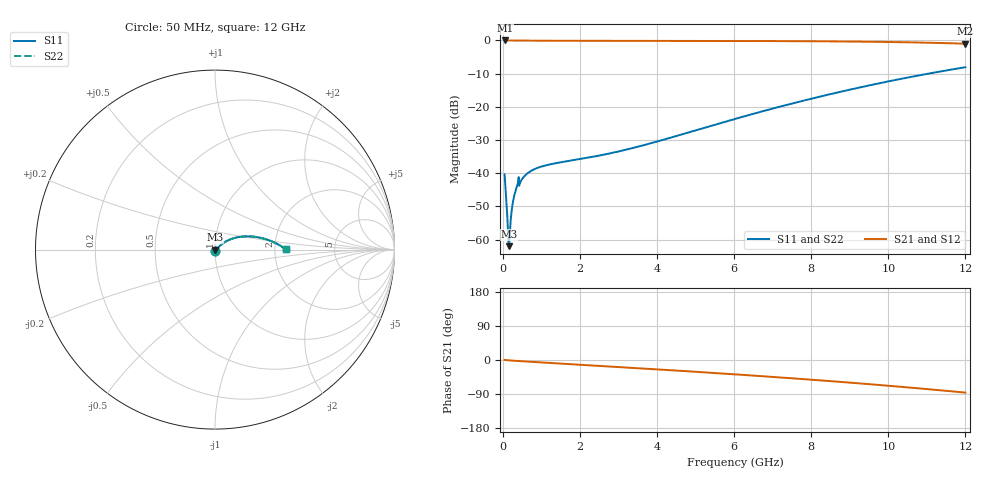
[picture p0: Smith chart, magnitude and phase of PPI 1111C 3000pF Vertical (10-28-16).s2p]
# GHz S MA R 50
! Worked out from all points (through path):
!   1601 points, 50 MHz to 12 GHz, reference 50 ohm
!   highest |S21| = 0.00 dB at 57.47 MHz (marker M1); lowest = -1.0 dB at 12 GHz (marker M2)
!   group delay of S21, straight-line fit = 19.5 ps
!   lowest |S11| = -62.0 dB at 162 MHz (marker M3), VSWR 1.00, Z = 50.1 - j0.0118 ohm
!   |S11| at or under -10 dB: start of sweep to 11.04 GHz
!   |S22| runs from -62.0 to -8.1 dB; largest |S21 - S12| = 0
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0.05  0.009595 -87.5  0.9996 0.3  0.9996 0.3  0.009595 -87.5
0.05746875  0.008105 -87.1  0.9996 0.1  0.9996 0.1  0.008105 -87.1
0.079875  0.005142 -85.3  0.9995 -0.2  0.9995 -0.2  0.005142 -85.3
0.1246875  0.001945 -73.5  0.9994 -0.6  0.9994 -0.6  0.001945 -73.5
0.139625  0.001272 -60.2  0.9993 -0.8  0.9993 -0.8  0.001272 -60.2
0.1620312  0.0007945 -8.6  0.9992 -0.9  0.9992 -0.9  0.0007945 -8.6
0.1844375  0.001223 36.8  0.999 -1.1  0.999 -1.1  0.001223 36.8
0.199375  0.001678 47.8  0.9989 -1.2  0.9989 -1.2  0.001678 47.8
0.2665938  0.003685 58.0  0.9981 -1.8  0.9981 -1.8  0.003685 58.0
0.3039375  0.004672 57.7  0.9976 -2.0  0.9976 -2.0  0.004672 57.7
0.3562187  0.005956 56.1  0.9968 -2.4  0.9968 -2.4  0.005956 56.1
0.438375  0.006753 48.6  0.9958 -2.9  0.9958 -2.9  0.006753 48.6
0.6026875  0.009499 44.7  0.9937 -4.0  0.9937 -4.0  0.009499 44.7
0.7894062  0.01124 38.7  0.9918 -5.1  0.9918 -5.1  0.01124 38.7
1.043344  0.01277 33.3  0.9901 -6.6  0.9901 -6.6  0.01277 33.3
2.044156  0.01647 28.0  0.9873 -12.6  0.9873 -12.6  0.01647 28.0
3.000156  0.0212 31.9  0.9861 -18.4  0.9861 -18.4  0.0212 31.9
4.038312  0.03037 36.8  0.985 -24.9  0.985 -24.9  0.03037 36.8
6.025  0.06568 37.8  0.9813 -37.9  0.9813 -37.9  0.06568 37.8
8.019156  0.1332 29.8  0.9721 -52.1  0.9721 -52.1  0.1332 29.8
10.01331  0.2422 16.8  0.9481 -68.0  0.9481 -68.0  0.2422 16.8
12  0.3947 0.2  0.8931 -86.1  0.8931 -86.1  0.3947 0.2
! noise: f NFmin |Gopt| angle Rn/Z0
0.05  0.0004232  0.8812  0.2986  0.0007718
1.372  0.01196  0.885  8.049  0.02246
2.701  0.01826  0.8558  15.75  0.02655
4.031  0.02307  0.8349  23.29  0.02833
5.36  0.02737  0.8211  30.59  0.02986
6.682  0.03147  0.8131  37.57  0.03153
8.012  0.03561  0.8097  44.28  0.03351
9.341  0.03991  0.8102  50.65  0.03589
10.67  0.04452  0.8139  56.67  0.03883
12  0.04956  0.8204  62.36  0.04248
